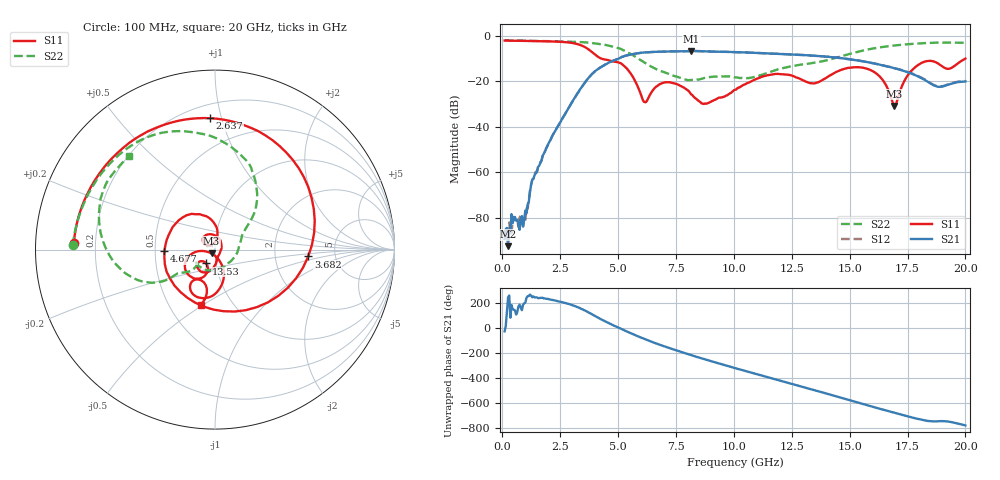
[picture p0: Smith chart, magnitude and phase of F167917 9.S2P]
!  2-Port S-parameters saved by WinCal
! VAR MeasName=S-Parameters (CALIBRATED_DATA) read from VNA (N5242A)
! VAR MeasDate=2016-11-22 9:00:08
! VAR NAME=F167917 9
! VAR FILENAME=F167917 9.S2P
! VAR DATE=2016-11-22 9:00:08
! VAR PHYS_PORTS=1,2
# Hz S DB R 50
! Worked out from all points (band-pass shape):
!   401 points, 100 MHz to 20 GHz, reference 50 ohm
!   highest |S21| = -6.65 dB at 8.159 GHz (marker M1); lowest = -92.5 dB at 249.2 MHz (marker M2)
!   |S21| within 3 dB of the highest: 5.096 GHz to 14.48 GHz (9.381 GHz wide, 95.9 % of centre)
!   lowest |S11| = -30.8 dB at 16.92 GHz (marker M3), VSWR 1.06, Z = 48.1 - j2.08 ohm
!   |S11| at or under -10 dB: 4.274 GHz to end of sweep
!   |S22| runs from -19.5 to -2.0 dB; largest |S21 - S12| = 0.004
!   S11 on the Smith chart (normalised r, x): 100 MHz: 0.12, +0.02; 2.637 GHz: 0.29, +0.92; 3.682 GHz: 3.14, -0.33; 4.677 GHz: 0.56, -0.01; 13.53 GHz: 0.90, -0.14; 20 GHz: 0.72, -0.49
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1e8  -2.09 177.3  -89.35 -27.7  -85.44 124.7  -2.02 178.3
2.4925e8  -2.10 173.3  -92.54 -119.0  -90.52 122.0  -2.05 175.9
9.955e8  -2.22 153.3  -76.85 -158.0  -80.90 -135.0  -2.18 164.4
1.34375e9  -2.28 143.3  -62.90 -109.8  -62.82 -110.2  -2.23 159.0
2.63725e9  -2.70 92.3  -35.60 -158.6  -35.63 -159.2  -2.46 137.1
3.43325e9  -4.28 28.2  -22.46 150.1  -22.48 150.0  -2.76 119.8
3.682e9  -5.66 -4.2  -19.02 127.0  -19.01 127.0  -2.95 113.6
4.12975e9  -9.20 -82.1  -14.61 81.1  -14.56 81.0  -3.49 101.5
4.677e9  -11.01 -178.1  -11.40 30.0  -11.36 29.6  -4.49 84.6
5.42325e9  -14.93 100.3  -8.47 -33.2  -8.47 -33.5  -7.32 58.0
6.1695e9  -29.22 119.2  -7.28 -91.6  -7.28 -91.8  -11.98 38.8
6.7665e9  -21.51 144.3  -6.97 -132.9  -6.97 -133.1  -15.19 28.7
8.1595e9  -25.78 50.5  -6.65 142.4  -6.67 142.3  -19.44 -55.3
1.005e10  -23.72 -83.6  -7.16 38.9  -7.17 39.0  -18.27 -148.9
1.199025e10  -16.83 -126.7  -7.98 -60.5  -7.93 -60.6  -14.52 -139.8
1.338325e10  -20.93 -129.3  -8.67 -132.1  -8.66 -131.8  -12.00 -147.6
1.35325e10  -20.77 -122.7  -8.79 -139.7  -8.77 -139.6  -11.77 -147.6
1.55225e10  -13.93 -144.4  -11.13 115.5  -11.08 115.4  -6.58 -159.2
1.67165e10  -25.00 -170.8  -13.64 53.8  -13.66 54.3  -4.51 -178.2
1.69155e10  -30.83 -131.1  -14.20 44.1  -14.12 44.4  -4.27 178.6
1.801e10  -12.48 -87.6  -18.13 -9.1  -17.95 -9.0  -3.34 161.4
2e10  -10.01 -104.5  -20.03 -58.6  -19.83 -58.7  -3.04 132.5
